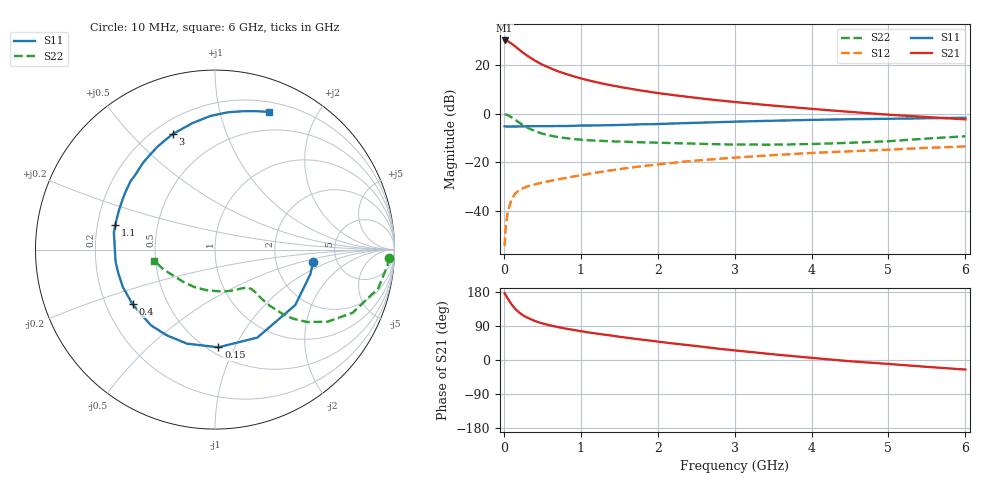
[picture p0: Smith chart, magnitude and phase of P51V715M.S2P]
! SIEMENS Small Signal Semiconductors
! BFP183
! Si NPN RF Bipolar Junction Transistor in SOT143
! VCE = 1.75 V  IC = 15 mA
! Common Emitter S-Parameters:  March  1996
# GHz  S  MA  R  50
!  f  S11  S21  S12  S22
! GHz  MAG  ANG  MAG  ANG  MAG  ANG  MAG  ANG
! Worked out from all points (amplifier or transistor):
!   36 points, 10 MHz to 6 GHz, reference 50 ohm
!   highest |S21| = 30.1 dB at 10 MHz (marker M1)
!   |S21| within 3 dB of that: start of sweep to 169.7 MHz
!   unconditionally stable (mu >= 1): 872.2 MHz to 5.657 GHz
!   at 250 MHz: K = 0.43, MSG = 27.8 dB, |S12| = -30.6 dB
!   at 1.4 GHz: K = 1.14, MAG = 15.1 dB, |S12| = -23.2 dB
!   at 6 GHz: K = 0.96, MSG = 5.6 dB, |S12| = -13.5 dB
!   S11 on the Smith chart (normalised r, x): 10 MHz: 3.31, -0.66; 150 MHz: 0.56, -0.86; 400 MHz: 0.31, -0.27; 1.1 GHz: 0.28, +0.11; 3 GHz: 0.27, +0.66; 6 GHz: 0.30, +1.42
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0.01  0.5512 -7.2  31.88 176.4  0.0019 80.8  0.973 -2.6
0.02  0.5487 -14.5  31.81 173.1  0.0039 84.7  0.9646 -5.4
0.05  0.5436 -34.7  30.89 162.2  0.0097 78.8  0.9349 -13.3
0.1  0.5439 -64.3  27.47 146.9  0.0172 64.1  0.8444 -24.6
0.15  0.5446 -88.0  23.9 134.5  0.0231 56.7  0.7454 -32.6
0.2  0.5468 -106.6  20.67 125.1  0.0269 52.1  0.6544 -38.1
0.25  0.5481 -119.6  17.84 117.8  0.0295 48.6  0.581 -41.5
0.3  0.5525 -130.3  15.7 112.2  0.0319 47.0  0.523 -43.5
0.4  0.5511 -146.4  12.43 103.1  0.0352 45.5  0.4413 -45.6
0.5  0.5542 -157.9  10.16 96.6  0.0384 44.7  0.3887 -46.4
0.6  0.5546 -166.0  8.665 91.4  0.0415 45.7  0.3553 -46.6
0.7  0.558 -173.0  7.442 87.0  0.0446 46.5  0.3319 -46.6
0.9  0.562 175.5  5.897 79.6  0.0511 48.0  0.3022 -47.2
1.1  0.5716 166.2  4.846 72.8  0.058 48.9  0.2845 -48.5
1.5  0.586 151.3  3.564 61.4  0.0722 49.4  0.2676 -53.1
1.8  0.6057 141.0  2.964 53.5  0.0836 48.9  0.2577 -58.2
2.2  0.6285 129.6  2.412 43.7  0.0978 46.4  0.248 -66.4
3  0.6854 110.2  1.738 25.4  0.1251 40.3  0.2319 -87.2
3.5  0.7159 100.1  1.463 15.1  0.1407 36.6  0.2309 -102.2
4.5  0.7685 84.6  1.087 -3.3  0.169 27.9  0.2521 -134.3
5.5  0.8041 73.6  0.853 -18.1  0.199 20.3  0.3083 -159.0
6  0.8236 68.7  0.765 -25.2  0.2117 15.6  0.3438 -169.7
